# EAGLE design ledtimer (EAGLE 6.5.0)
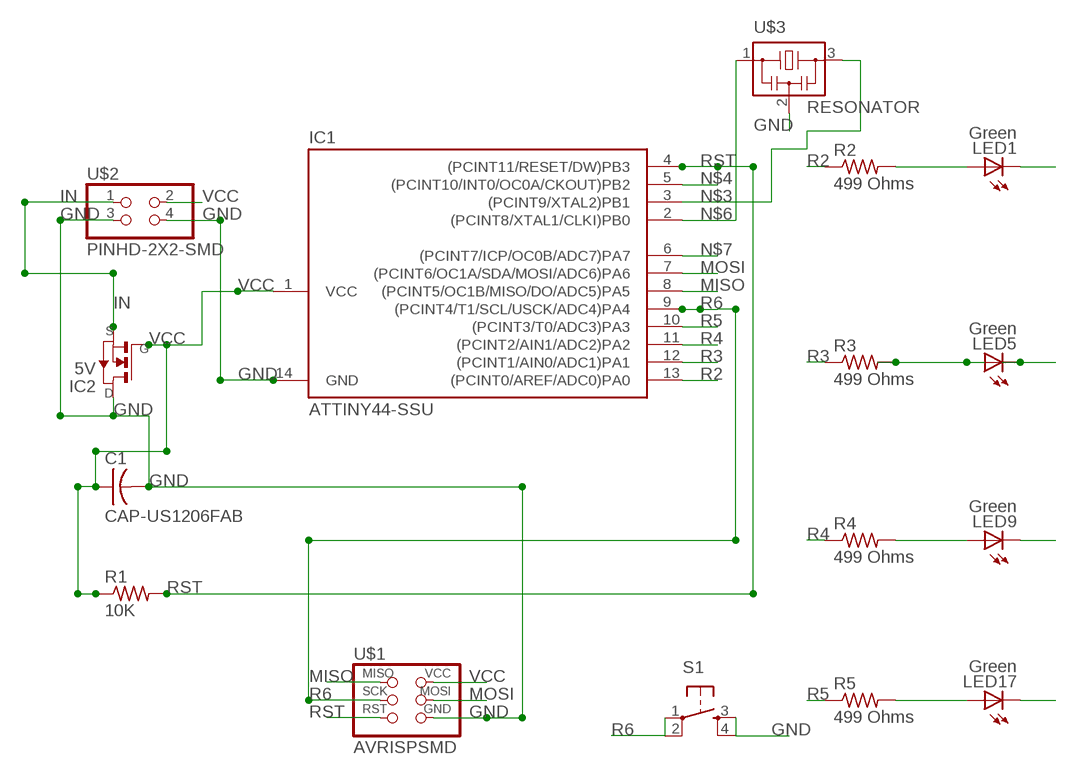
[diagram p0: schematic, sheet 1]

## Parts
C1  CAP-US1206FAB  [C1206FAB]
IC1  ATTINY44-SSU  [SOIC14]
IC2  5V  NMOSFETSOT23  [SOT-23]
LED1  Green  LEDSML1206  [SML1206]
LED5  Green  LEDSML1206  [SML1206]
LED9  Green  LEDSML1206  [SML1206]
LED17  Green  LEDSML1206  [SML1206]
R1  10K  RES-US1206FAB  [R1206FAB]
R2  499 Ohms  RES-US1206FAB  [R1206FAB]
R3  499 Ohms  RES-US1206FAB  [R1206FAB]
R4  499 Ohms  RES-US1206FAB  [R1206FAB]
R5  499 Ohms  RES-US1206FAB  [R1206FAB]
S1  6MM_SWITCH6MM_SWITCH  [6MM_SWITCH]
U$1  AVRISPSMD  [2X03SMD]
U$2  PINHD-2X2-SMD  [2X02SMD]
U$3  RESONATOR  [EFOBM]

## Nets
GND: C1.2 IC1.14(GND) IC2.1(D) LED1.C LED5.C LED9.C LED17.C S1.3(S) S1.4(S1) U$1.6(GND) U$2.3 U$2.4 U$3.2
IN: IC2.2(S) U$2.1
MISO: IC1.8((PCINT5/OC1B/MISO/DO/ADC5)PA5) U$1.1(MISO)
MOSI: IC1.7((PCINT6/OC1A/SDA/MOSI/ADC6)PA6) U$1.4(MOSI)
N$1: LED1.A R2.2
N$2: LED5.A R3.2
N$3: IC1.3((PCINT9/XTAL2)PB1) U$3.3
N$4: IC1.5((PCINT10/INT0/OC0A/CKOUT)PB2)
N$5: LED9.A R4.2
N$6: IC1.2((PCINT8/XTAL1/CLKI)PB0) U$3.1
N$7: IC1.6((PCINT7/ICP/OC0B/ADC7)PA7)
N$8: LED17.A R5.2
R2: IC1.13((PCINT0/AREF/ADC0)PA0) R2.1
R3: IC1.12((PCINT1/AIN0/ADC1)PA1) R3.1
R4: IC1.11((PCINT2/AIN1/ADC2)PA2) R4.1
R5: IC1.10((PCINT3/T0/ADC3)PA3) R5.1
R6: IC1.9((PCINT4/T1/SCL/USCK/ADC4)PA4) S1.1(P) S1.2(P1) U$1.3(SCK)
RST: IC1.4((PCINT11/RESET/DW)PB3) R1.2 U$1.5(RST)
VCC: C1.1 IC1.1(VCC) IC2.3(G) R1.1 U$1.2(VCC) U$2.2

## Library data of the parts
C1 = fab2:CAP-US
IC1 = fab2:ATTINY44
IC2 = fab:NMOSFET: MOS FET
LED1 LED5 LED9 LED17 = led:LED: LED
R1-R5 = fab2:RES-US: Resistor (US Symbol)
S1 = fab:6MM_SWITCH: OMRON SWITCH
U$1 = fab2:AVRISP
U$2 = fab:PINHD-2X2-SMD
U$3 = fab:RESONATOR

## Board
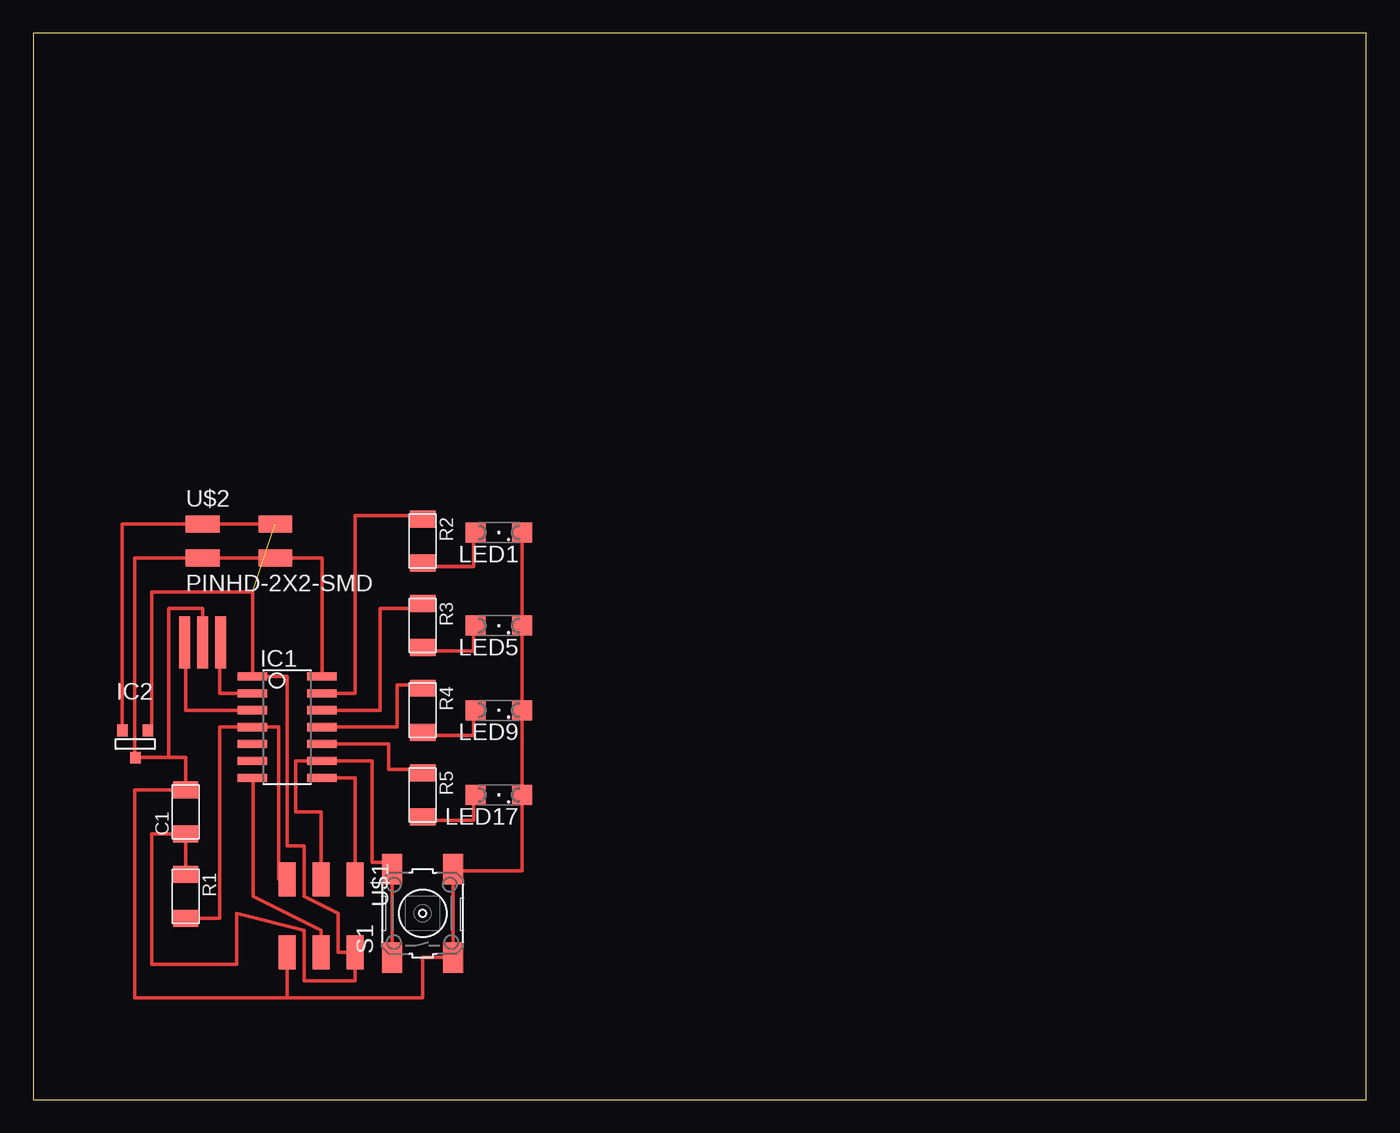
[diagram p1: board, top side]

Size 100 x 80 mm. Coordinates in mm from the lower left corner, seen from the top.
Outline: 0,0 100,0 100,80 0,80 0,0
Copper layers (1*16): Top 0.035mm / dielectric 1.5mm / Bottom 0.035mm
Design rules "default *": minimum track width 10mil, minimum drill 24mil, track to track 16mil, track to pad 16mil, pad to pad 8mil, via to via 8mil, smd to smd 8mil, copper to edge 40mil, drill to drill 8mil, minimum pad ring 10mil, minimum via ring 8mil, stop-mask expansion 4mil, vias tented up to drill 0mil, thermal gap 10mil

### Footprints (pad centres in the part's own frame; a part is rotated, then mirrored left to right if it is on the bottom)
C1206FAB = smd 1.27 x 1.905: 1 -1.651,0; 2 1.651,0
SOIC14 = smd 0.61 x 2.21: 1 -3.81,-2.603; 2 -2.54,-2.603; 3 -1.27,-2.603; 4 0,-2.603; 5 1.27,-2.603; 6 2.54,-2.603; 7 3.81,-2.603; 8 3.81,2.603; 9 2.54,2.603; 10 1.27,2.603; 11 0,2.603; 12 -1.27,2.603; 13 -2.54,2.603; 14 -3.81,2.603
SOT-23 = smd 0.787 x 0.889: 1 0.025,-1.016; 2 -0.94,1.016; 3 0.991,1.016
SML1206 = smd 1.5 x 1.5: A 1.75,0; C -1.75,0
R1206FAB = smd 1.27 x 1.905: 1 -1.651,0; 2 1.651,0
6MM_SWITCH = smd 2.286 x 1.524: 1 -3.302,2.286; 2 3.302,2.286; 3 -3.302,-2.286; 4 3.302,-2.286
2X03SMD = smd 2.54 x 1.27: 1 -2.54,2.54; 2 2.92,2.54; 3 -2.54,0; 4 2.92,0; 5 -2.54,-2.54; 6 2.92,-2.54
2X02SMD = smd 2.54 x 1.27: 1 -2.54,1.27; 2 2.92,1.27; 3 -2.54,-1.27; 4 2.92,-1.27
EFOBM = smd 0.8 x 3.9: 1 -1.35,0; 2 0,0; 3 1.35,0

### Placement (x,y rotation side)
C1  11.43,21.59 90 top
IC1  19.05,27.94 270 top
IC2  7.62,26.67 0 top
LED1  34.92,42.55 180 top
LED5  34.92,35.56 180 top
LED9  34.92,29.21 180 top
LED17  34.92,22.86 180 top
R1  11.43,15.24 270 top
R2  29.21,41.91 270 top
R3  29.21,35.56 270 top
R4  29.21,29.21 270 top
R5  29.21,22.86 270 top
S1  29.21,13.97 90 top
U$1  21.59,13.97 270 top
U$2  15.24,41.91 0 top
U$3  12.7,34.29 180 top

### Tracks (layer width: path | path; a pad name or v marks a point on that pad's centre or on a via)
GND
  Top 0.254: IC1.14 21.65,40.64 U$2.4 U$2.3 7.62,40.64 7.62,25.65 IC2.1 10.16,25.65 | 31.5,17.14 S1.3 29.21,10.67 29.21,7.62 19.05,7.62 | 10.16,25.65 11.43,25.65 C1.2 7.62,23.24 7.62,7.62 19.05,7.62 | U$3.2 12.7,36.83 10.16,36.83 10.16,25.65 | 19.05,11.43 U$1.6 19.05,7.62 | LED17.C LED9.C LED5.C LED1.C | LED17.C 36.83,22.86 | 31.5,17.14 S1.4 | 31.5,17.14 36.67,17.14 LED17.C
IN
  Top 0.254: U$2.1 6.68,43.18 IC2.2
MISO
  Top 0.254: U$1.1 24.13,24.13 IC1.8
MOSI
  Top 0.254: U$1.4 21.59,12.7 16.51,15.24 16.51,24.13 IC1.7
N$1
  Top 0.254: LED1.A 33.02,42.55 33.02,40.01 29.21,40.01 R2.2
N$2
  Top 0.254: LED5.A 33.02,35.56 33.02,33.66 29.21,33.66 R3.2
N$3
  Top 0.254: U$3.3 11.43,34.29 11.43,29.21 IC1.3
N$5
  Top 0.254: LED9.A 33.02,29.21 33.02,27.3 29.21,27.3 R4.2
N$6
  Top 0.254: IC1.2 13.97,30.48 13.97,33.02 14.05,33.02 U$3.1
N$8
  Top 0.254: LED17.A 33.02,22.86 33.02,20.95 29.21,20.95 R5.2
R2
  Top 0.254: IC1.13 24.13,30.48 24.13,43.81 29.21,43.81 R2.1
R3
  Top 0.254: IC1.12 26.04,29.21 26.04,36.83 29.21,36.83 R3.1
R4
  Top 0.254: 29.21,30.48 R4.1 29.21,31.11 27.3,31.11 27.3,27.94 IC1.11
R5
  Top 0.254: IC1.10 26.67,26.67 26.67,24.77 29.21,24.77 R5.1
R6
  Top 0.254: U$1.3 21.59,21.59 19.68,21.59 19.68,25.4 IC1.9 25.4,25.4 25.4,17.78 26.92,17.78 S1.2 S1.1
RST
  Top 0.254: R1.2 13.97,13.59 13.97,27.94 IC1.4 18.41,27.94 18.41,16.51 U$1.5
VCC  (1 unrouted)
  Top 0.254: R1.1 C1.1 8.89,19.94 8.89,10.16 15.24,10.16 15.24,13.97 20.32,12.7 20.32,8.89 24.13,8.89 U$1.2 22.86,11.05 22.86,13.97 20.32,15.24 20.32,19.05 19.05,19.05 19.05,31.75 IC1.1 16.45,36.83 16.45,38.1 8.89,38.1 8.89,27.69 IC2.3 | U$2.2 12.7,43.18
